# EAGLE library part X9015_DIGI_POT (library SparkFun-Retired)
Digital pot- up/down/increment control only Prototype: IC-08072 no stock, old part (2008-2010)
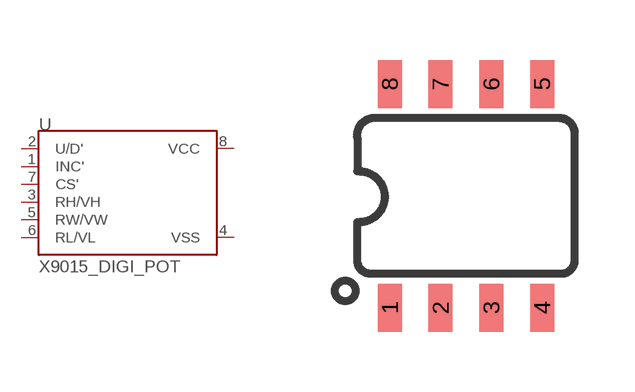
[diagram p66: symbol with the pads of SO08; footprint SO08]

Designator prefix -

## X9015_DIGI_POTS  [SO08]
1  INC'
2  U/D'
3  RH/VH
4  VSS  pwr
5  RW/VW
6  RL/VL
7  CS'
8  VCC  pwr

## Footprint SO08 (pad centres in mm)
SOIC, 0.15 inch width
smd 0.6 x 1.2: 1 -1.905,-2.8; 2 -0.635,-2.8; 3 0.635,-2.8; 4 1.905,-2.8; 5 1.905,2.8; 6 0.635,2.8; 7 -0.635,2.8; 8 -1.905,2.8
